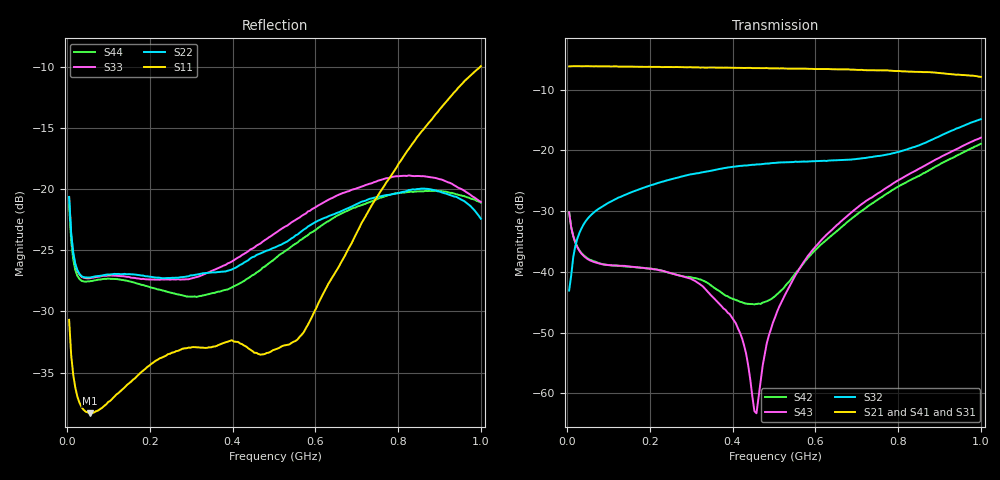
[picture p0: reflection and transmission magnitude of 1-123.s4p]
!Vector Network Analyzer,NA7684A,8000025053,DSP: 1.0.1
!Date: 2021-10-28 16:49
!Data & Calibration Information:
!Freq	S11:SOLT4(ON)	S12:SOLT4(ON)	S13:SOLT4(ON)	S14:SOLT4(ON)
!	S21:SOLT4(ON)	S22:SOLT4(ON)	S23:SOLT4(ON)	S24:SOLT4(ON)
!	S31:SOLT4(ON)	S32:SOLT4(ON)	S33:SOLT4(ON)	S34:SOLT4(ON)
!	S41:SOLT4(ON)	S42:SOLT4(ON)	S43:SOLT4(ON)	S44:SOLT4(ON)
# Hz S dB R 50
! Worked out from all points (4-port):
!   201 points, 5 MHz to 1 GHz, reference 50 ohm
!   strongest paths, dB at 5 MHz, 253.8 MHz, 502.5 MHz, 751.2 MHz, 1 GHz:
!     S21: -6.2, -6.3, -6.5, -6.8, -7.9
!     S41: -6.2, -6.3, -6.6, -7.0, -8.2
!     S31: -6.2, -6.3, -6.6, -7.0, -8.2
!     S32: -43.1, -24.7, -22.1, -20.9, -14.9
!     S43: -30.2, -40.3, -47.5, -27.1, -17.9
!     S42: -30.2, -40.3, -44.0, -28.1, -18.9
!   lowest |S11| = -38.3 dB at 54.75 MHz (marker M1), VSWR 1.02, Z = 50.2 + j1.2 ohm
!   |S11| at or under -10 dB: start of sweep to 998 MHz
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5000000  -30.68 120.6  -6.19 0.5  -6.22 0.6  -6.21 0.6
         -6.19 0.1  -20.63 137.2  -43.09 39.7  -30.16 -42.9
         -6.20 0.0  -43.09 40.1  -20.65 137.1  -30.18 -42.9
         -6.24 -0.1  -30.18 -43.1  -30.20 -42.7  -21.26 137.4
5.475e7  -38.33 82.0  -6.18 -11.9  -6.19 -12.0  -6.17 -12.0
         -6.17 -12.3  -27.22 172.9  -30.84 45.2  -37.86 -26.3
         -6.19 -12.5  -30.88 45.4  -27.28 172.9  -38.11 -22.6
         -6.21 -12.7  -37.99 -26.3  -38.10 -22.3  -27.53 172.5
3.28375e8  -32.96 -32.1  -6.36 -74.2  -6.39 -75.0  -6.37 -75.3
           -6.36 -74.5  -26.87 -168.9  -23.58 24.5  -41.53 -64.0
           -6.42 -75.4  -23.61 24.7  -27.00 -163.7  -43.01 -26.2
           -6.41 -75.8  -41.44 -65.3  -42.41 -28.4  -28.69 -169.7
4.57725e8  -33.38 -91.4  -6.45 -104.7  -6.52 -105.8  -6.49 -106.2
           -6.46 -104.9  -25.38 -160.8  -22.41 16.2  -45.13 -137.5
           -6.53 -106.3  -22.33 16.5  -24.61 -155.1  -56.46 60.6
           -6.52 -107.0  -45.29 -137.7  -63.29 58.0  -26.82 -153.9
4.97525e8  -33.17 -120.1  -6.50 -114.4  -6.57 -115.6  -6.57 -115.9
           -6.51 -114.8  -24.81 -159.4  -22.17 14.0  -44.13 -172.7
           -6.59 -116.3  -22.09 14.0  -23.71 -155.2  -47.34 99.2
           -6.57 -116.7  -44.27 -170.5  -48.38 108.2  -25.83 -151.9
5.9205e8  -30.42 167.1  -6.62 -137.9  -6.67 -139.6  -6.66 -140.1
          -6.60 -138.4  -22.85 -163.4  -21.89 10.8  -36.95 136.0
          -6.69 -140.1  -21.81 10.8  -21.63 -159.7  -36.58 101.8
          -6.65 -140.9  -36.99 134.8  -36.51 104.7  -23.51 -153.8
1e9  -9.93 -12.2  -7.93 100.8  -8.25 97.6  -8.14 97.6
     -7.91 100.2  -22.41 136.8  -14.82 5.0  -18.85 20.0
     -8.24 96.9  -14.87 5.5  -21.04 153.9  -17.95 17.5
     -8.16 97.0  -18.92 20.1  -17.92 16.5  -21.10 163.5
